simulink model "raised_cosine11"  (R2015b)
settings: Solver=VariableStepAuto  StartTime=0.0  StopTime=5  RelTol=1e-3
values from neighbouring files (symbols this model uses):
  hrc = hrc/sum(hrc)    [raised_cosine_1.m]    (also in raised_cosine_2.m = rcosdesign(alpha, n_symb, Tsymb/Ts,'normal'); raised_cosine_3.m = rcosdesign(alpha, n_symb, Tsymb/Ts))
  k_norm = 1/(fs*sum(hamming(n_fft).^2))    [raised_cosine_1.m]    (also in raised_cosine_2.m)
  n_fft = 256    [raised_cosine_1.m]    (also in raised_cosine_2.m; raised_cosine_3.m)
  n_symb = 4    [raised_cosine_1.m]    (also in raised_cosine_2.m = 8; raised_cosine_3.m = 6)
  ns = length(ys(:,1))    [hilbert_filter_1.m]    (also in raised_cosine_1.m = 5; raised_cosine_2.m = 5; raised_cosine_3.m = 5)
  Ts = 1/fs    (= 0.001)    [abtast_fir_1.m]    (also in abtast_fir_2.m; abtast_fir_3.m; abtast_fir_4.m; hilbert_filter_1.m)
  Tsymb = ns*Ts    (= 0.005)    [raised_cosine_1.m]    (also in raised_cosine_2.m; raised_cosine_3.m)
undefined symbols (not defined in the file or in its folder): dBWatt, Fs, get, Hz
libraries: dspstat3 x3, dspsigops x3, dspspect3 x2, dspsnks4 x1

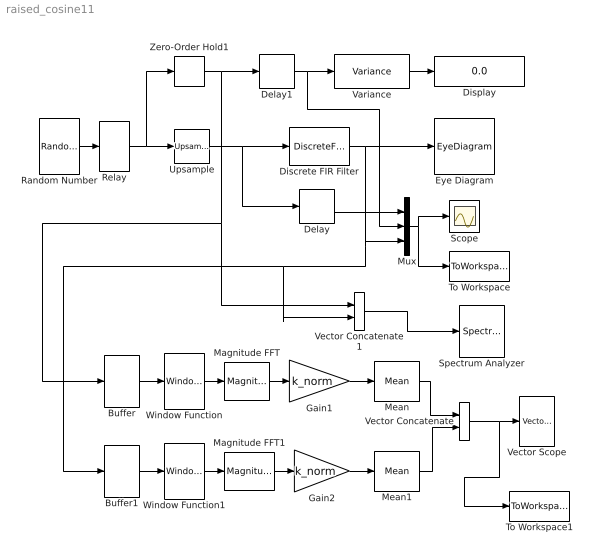
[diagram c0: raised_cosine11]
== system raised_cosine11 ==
  Buffer : Buffer  N=n_fft  V=n_fft/2  TreatMby1Signals=One channel  OutputFrames=off
  Buffer1 : Buffer  N=n_fft  V=n_fft/2  TreatMby1Signals=One channel  OutputFrames=off
  Delay : Delay  DelayLength=n_symb*Tsymb/Ts  SampleTime=Ts
  Delay1 : Delay  DelayLength=n_symb*Tsymb/Ts  SampleTime=Ts
  Discrete FIR Filter : DiscreteFir  Coefficients=hrc/max(hrc)  SampleTime=Ts
  Display : Display
  Eye Diagram : EyeDiagram
  Gain1 : Gain  Gain=k_norm
  Gain2 : Gain  Gain=k_norm
  Magnitude FFT : dspspect3/Magnitude FFT  mag_or_magsq=Magnitude squared  FFTImplementation=Auto  fftLenInherit=on  fftsize=256  WrapInput=on
  Magnitude FFT1 : dspspect3/Magnitude FFT  mag_or_magsq=Magnitude squared  FFTImplementation=Auto  fftLenInherit=on  fftsize=256  WrapInput=on
  Mean : dspstat3/Mean  run=on  reset_popup=None  directionMode=Each column  dimension=1  roiEnable=off  roiType=Rectangles  roiPortion=Entire ROI  roiOutput=Individual statistics for each ROI  roiFlag=off  outputDataTypeStr=Inherit: Same as accumulator  outputLastDataTypeStr=Inherit: Same as accumulator  outputMin=[]  outputMax=[]  roundingMode=Floor  overflowMode=off
  Mean1 : dspstat3/Mean  run=on  reset_popup=None  directionMode=Each column  dimension=1  roiEnable=off  roiType=Rectangles  roiPortion=Entire ROI  roiOutput=Individual statistics for each ROI  roiFlag=off  outputDataTypeStr=Inherit: Same as accumulator  outputLastDataTypeStr=Inherit: Same as accumulator  outputMin=[]  outputMax=[]  roundingMode=Floor  overflowMode=off
  Mux : Mux  Inputs=3
  Random Number : RandomNumber  SampleTime=Tsymb
  Relay : Relay  OffOutputValue=-1
  Scope : Scope
  Spectrum Analyzer : SpectrumAnalyzer
  To Workspace : ToWorkspace  VariableName=y  SaveFormat=Timeseries  SampleTime=Ts
  To Workspace1 : ToWorkspace  VariableName=psd_y  SaveFormat=Timeseries  SampleTime=Ts
  Upsample : dspsigops/Upsample  N=ns  phase=0  RateOptions=Allow multirate processing  ic=0  mode=Unused parameter value
  Variance : dspstat3/Variance  run=on  reset_popup=None  directionMode=Each column  dimension=1  roiEnable=off  roiType=Rectangles  roiPortion=Entire ROI  roiOutput=Individual statistics for each ROI  roiFlag=off  roundingMode=Floor  overflowMode=off
  Vector Concatenate : Concatenate  Mode=Multidimensional array  ConcatenateDimension=2
  Vector Concatenate1 : Concatenate  Mode=Multidimensional array  ConcatenateDimension=2
  Vector Scope : dspsnks4/Vector Scope  ScopeProperties=on  Domain=Frequency  HorizSpan=1  DisplayProperties=off  AxisGrid=on  Memory=off  FrameNumber=on  AxisLegend=off  AxisZoom=off  OpenScopeAtSimStart=on  OpenScopeImmediately=off  FigPos=get(0,'defaultfigureposition')  AxisProperties=off  XUnits=Hertz  XRange=[-Fs/2...Fs/2]  InheritXIncr=off  XIncr=Ts  XLabel=Time  XLimit=User-defined  XMin=-500  XMax=500  XStart=0  YUnits=dB  YLabel=dBWatt/Hz  LineProperties=off  XAxisParamsVer=6.9
  Window Function : dspsigops/Window Function  winmode=Apply window to input  wintype=Hamming  sampmode=Continuous  samptime=1  N=64  Rs=50  beta=10  winsamp=Symmetric  UserWindow=hamming  OptParams=off  UserParams={'symmetric'}  dataType=double  isSigned=on  wordLen=16  udDataType=sfix(16)  fracBitsMode=Best precision  numFracBits=15  roundingMode=Floor  overflowMode=off  numSidelobes=4  sidelobeLevel=-30
  Window Function1 : dspsigops/Window Function  winmode=Apply window to input  wintype=Hamming  sampmode=Continuous  samptime=1  N=64  Rs=50  beta=10  winsamp=Symmetric  UserWindow=hamming  OptParams=off  UserParams={'symmetric'}  dataType=double  isSigned=on  wordLen=16  udDataType=sfix(16)  fracBitsMode=Best precision  numFracBits=15  roundingMode=Floor  overflowMode=off  numSidelobes=4  sidelobeLevel=-30
  Zero-Order Hold1 : ZeroOrderHold  SampleTime=Ts
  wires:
  Random Number/1 -> Relay/1
  Upsample/1 -> Delay/1, Discrete FIR Filter/1
  Mux/1 -> Scope/1, To Workspace/1
  Delay/1 -> Mux/1
  Relay/1 -> Zero-Order Hold1/1, Upsample/1
  Delay1/1 -> Mux/2, Variance/1
  Buffer/1 -> Window Function/1
  Magnitude FFT/1 -> Gain1/1
  Gain1/1 -> Mean/1
  Discrete FIR Filter/1 -> Vector Concatenate1/2, Buffer1/1, Mux/3, Eye Diagram/1
  Buffer1/1 -> Window Function1/1
  Gain2/1 -> Mean1/1
  Magnitude FFT1/1 -> Gain2/1
  Mean1/1 -> Vector Concatenate/2
  Mean/1 -> Vector Concatenate/1
  Vector Concatenate/1 -> To Workspace1/1, Vector Scope/1
  Variance/1 -> Display/1
  Vector Concatenate1/1 -> Spectrum Analyzer/1
  Window Function/1 -> Magnitude FFT/1
  Window Function1/1 -> Magnitude FFT1/1
  Zero-Order Hold1/1 -> Vector Concatenate1/1, Buffer/1, Delay1/1
